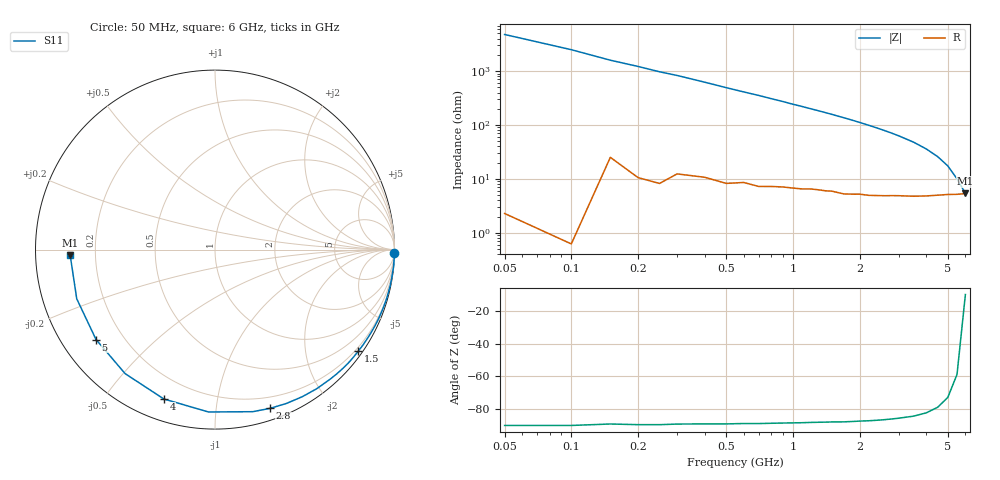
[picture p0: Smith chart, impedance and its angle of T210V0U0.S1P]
! SIEMENS Discrete & RF Semiconductors
! BAS70-04W
! Si Schottky Diode in SOT323
! VR = 10 V
! S-Parameters:  November  1997
# GHz  S  MA  R  50
!  f  S11
! GHz  MAG  ANG
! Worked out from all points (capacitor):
!   34 points, 50 MHz to 6 GHz, reference 50 ohm
!   read as one part to ground: C = 667 fF near 50 MHz
!   lowest |Z| = 5.41 ohm at 6 GHz (marker M1)
!   S11 on the Smith chart (normalised r, x): 50 MHz: 0, -95; 1.5 GHz: 0.12, -3.14; 2.8 GHz: 0.10, -1.40; 4 GHz: 0.10, -0.71; 5 GHz: 0.10, -0.33; 6 GHz: 0.11, -0.02
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0.05  1 -1.2
0.25  0.9991 -5.9
0.3  0.9982 -6.9
0.4  0.9972 -9.2
0.5  0.9966 -11.6
0.7  0.9943 -16.1
0.8  0.9926 -18.5
0.9  0.9908 -20.8
1  0.989 -23.3
1.1  0.9873 -25.6
1.3  0.9829 -30.4
1.4  0.981 -32.8
1.5  0.9785 -35.3
1.6  0.9768 -37.9
1.7  0.9752 -40.4
1.9  0.9693 -45.6
2  0.9657 -48.3
2.2  0.9603 -53.8
2.4  0.9531 -59.3
2.6  0.9451 -65.1
2.8  0.9362 -70.9
3  0.9272 -76.9
3.5  0.9054 -92.3
4  0.8797 -108.9
4.5  0.8534 -125.9
5  0.8309 -142.9
5.5  0.8176 -160.4
6  0.8075 -177.8
